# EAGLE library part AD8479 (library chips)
a very high common mode input opamp
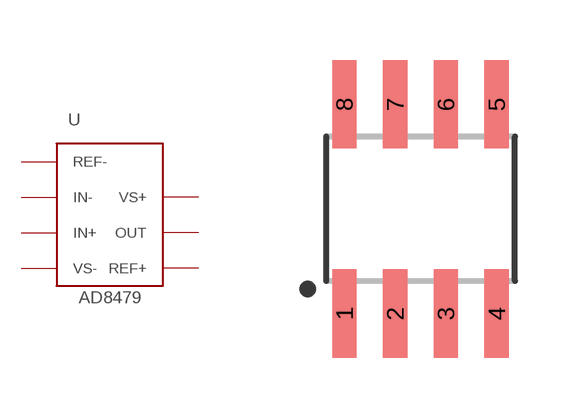
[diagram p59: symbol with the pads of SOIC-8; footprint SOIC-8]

Designator prefix -

## AD8479 (DIGIKEY: AD8479ARZ-ND)  [SOIC-8]
1  REF-
2  IN-
3  IN+
4  VS-
5  REF+
6  OUT
7  VS+

## Footprint SOIC-8 (pad centres in mm)
smd 0.61 x 2.21: 1 -1.905,-2.616; 2 -0.635,-2.616; 3 0.635,-2.616; 4 1.905,-2.616; 5 1.905,2.616; 6 0.635,2.616; 7 -0.635,2.616; 8 -1.905,2.616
